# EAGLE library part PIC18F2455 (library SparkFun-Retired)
PIC18F2455-I/SO Retired: IC-08246
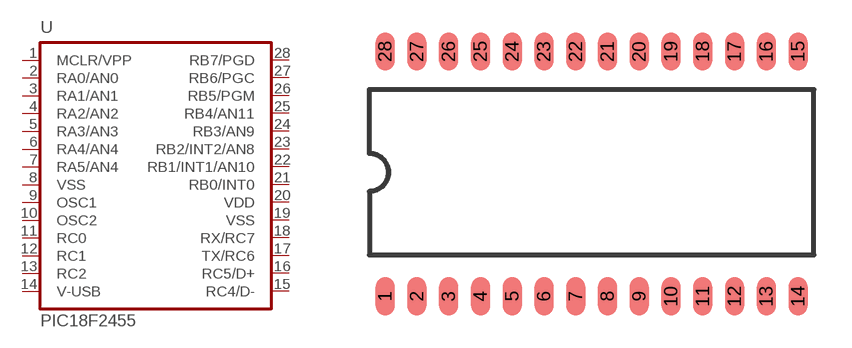
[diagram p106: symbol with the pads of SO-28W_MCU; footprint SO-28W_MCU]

Designator prefix -

## PIC18F2455SMD  [SO-28W_MCU]
1  MCLR/VPP
2  RA0/AN0
3  RA1/AN1
4  RA2/AN2
5  RA3/AN3
6  RA4/AN4
7  RA5/AN4
8  VSS  pwr
9  OSC1
10  OSC2
11  RC0
12  RC1
13  RC2
14  V-USB
15  RC4/D-
16  RC5/D+
17  TX/RC6
18  RX/RC7  in
19  VSS  pwr
20  VDD  pwr
21  RB0/INT0
22  RB1/INT1/AN10
23  RB2/INT2/AN8
24  RB3/AN9
25  RB4/AN11
26  RB5/PGM
27  RB6/PGC
28  RB7/PGD

## Footprint SO-28W_MCU (pad centres in mm)
Small Outline Wide Plastic Gull Wing 300-mil body, package type SO
smd 0.762 x 1.524: 1 -8.255,-4.953; 2 -6.985,-4.953; 3 -5.715,-4.953; 4 -4.445,-4.953; 5 -3.175,-4.953; 6 -1.905,-4.953; 7 -0.635,-4.953; 8 0.635,-4.953; 9 1.905,-4.953; 10 3.175,-4.953; 11 4.445,-4.953; 12 5.715,-4.953; 13 6.985,-4.953; 14 8.255,-4.953; 15 8.255,4.826; 16 6.985,4.826; 17 5.715,4.826; 18 4.445,4.826; 19 3.175,4.826; 20 1.905,4.826; 21 0.635,4.826; 22 -0.635,4.826; 23 -1.905,4.826; 24 -3.175,4.826; 25 -4.445,4.826; 26 -5.715,4.826; 27 -6.985,4.826; 28 -8.255,4.826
